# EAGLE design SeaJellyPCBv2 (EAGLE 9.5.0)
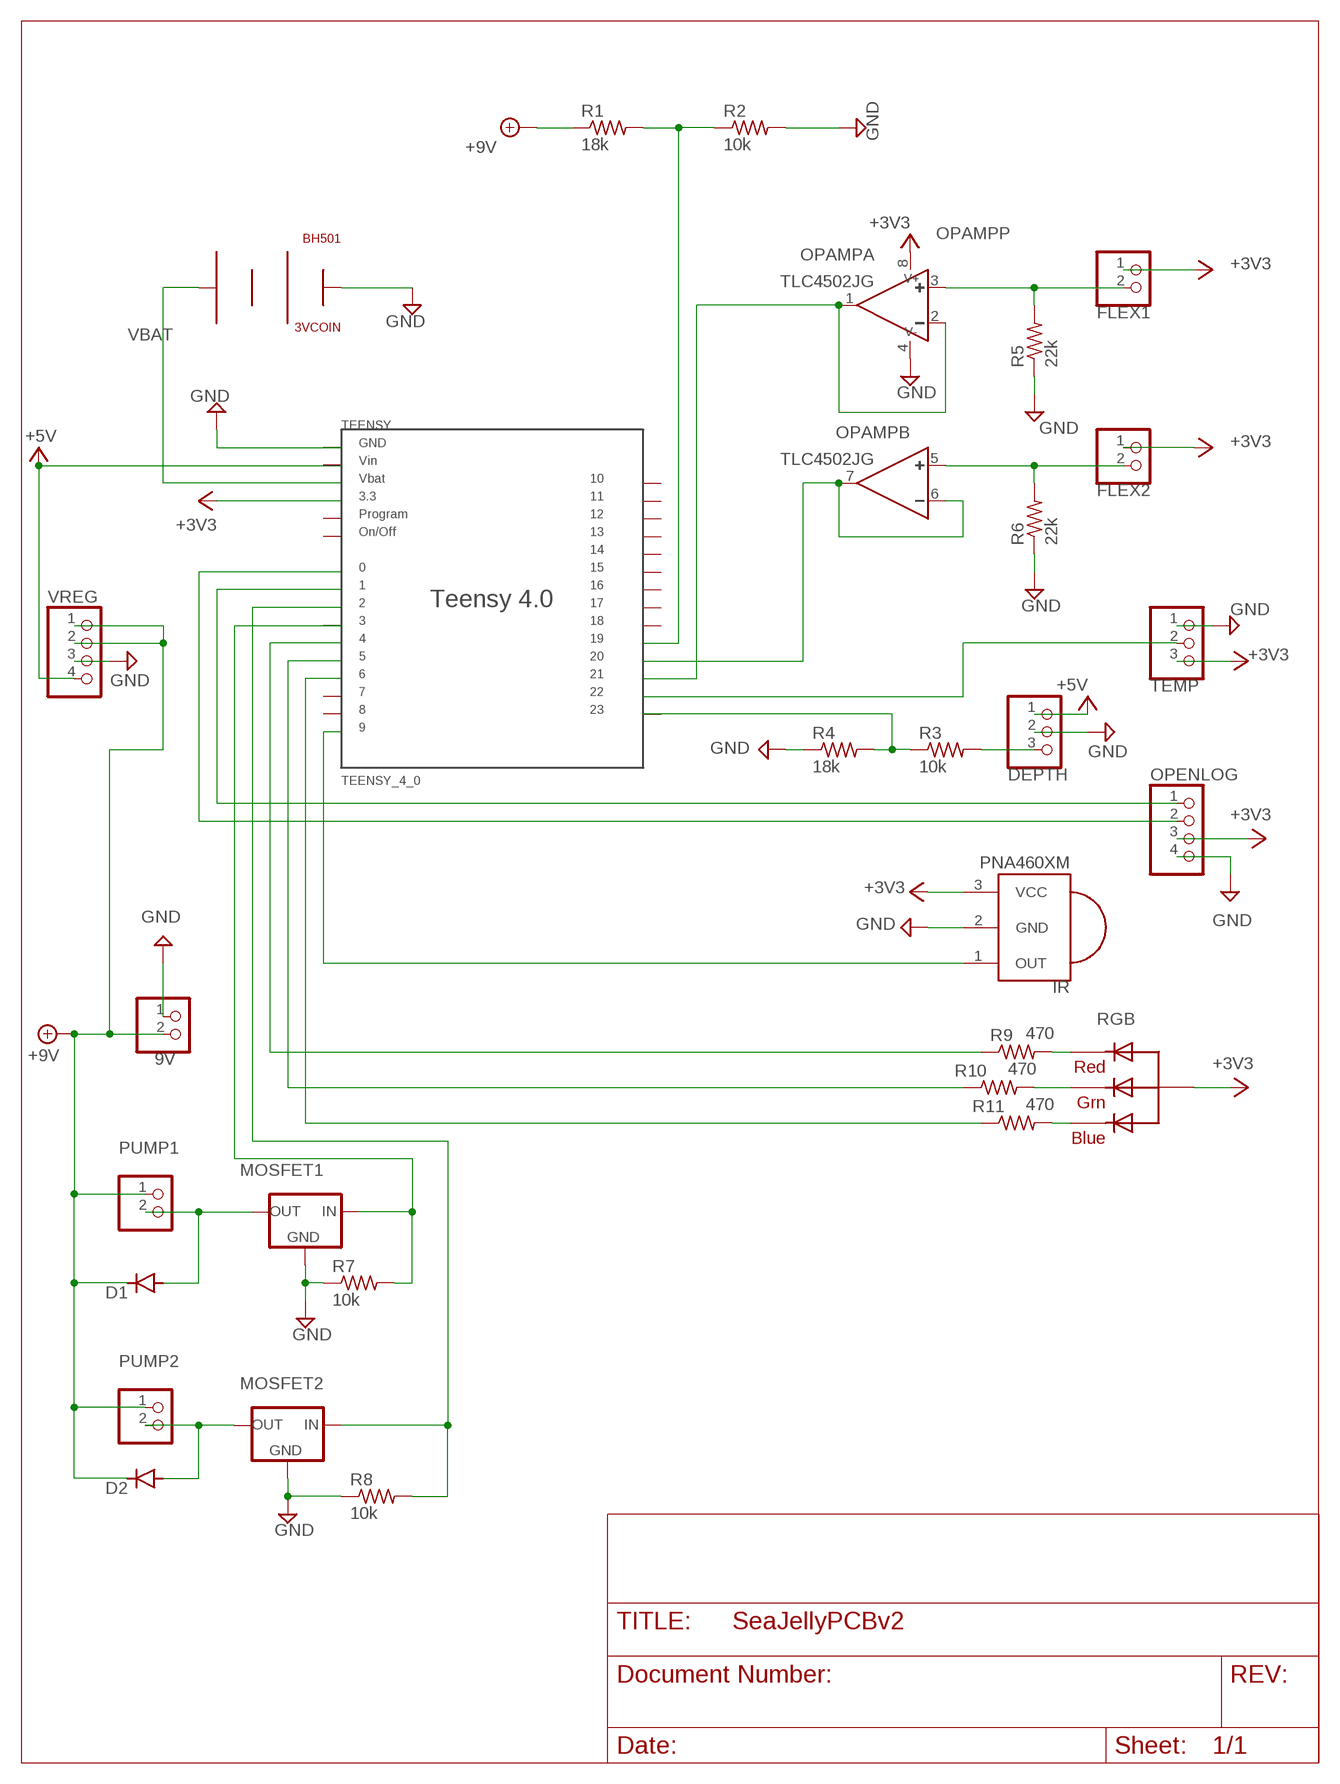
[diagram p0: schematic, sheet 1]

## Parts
3VCOIN  BH501  [BH501]
9V  PINHD-1X2  [1X02]
D1  DIODE-D-7.5  [D-7.5]
D2  DIODE-D-7.5  [D-7.5]
DEPTH  PINHD-1X3  [1X03]
FLEX1  PINHD-1X2  [1X02]
FLEX2  PINHD-1X2  [1X02]
IR  PNA460XM  [PNA460XM]
MOSFET1  MCP1700INLINE  [TO92-INLINE]
MOSFET2  MCP1700INLINE  [TO92-INLINE]
OPAMP  TLC4502JG  [DIL08]
OPENLOG  PINHD-1X4  [1X04]
PUMP1  PINHD-1X2  [1X02]
PUMP2  PINHD-1X2  [1X02]
R1  18k  R-US_0411/3V  [0411V]
R2  10k  R-US_0411/3V  [0411V]
R3  10k  R-US_0411/3V  [0411V]
R4  18k  R-US_0411/3V  [0411V]
R5  22k  R-US_0411/3V  [0411V]
R6  22k  R-US_0411/3V  [0411V]
R7  10k  R-US_0411/3V  [0411V]
R8  10k  R-US_0411/3V  [0411V]
R9  470  R-US_0411/3V  [0411V]
R10  470  R-US_0411/3V  [0411V]
R11  470  R-US_0411/3V  [0411V]
RGB  RGBLED_CA-5MM  [LED5MMRGB]
TEENSY  TEENSY_4_0  [TEENSY_4_0]
TEMP  PINHD-1X3  [1X03]
VREG  PINHD-1X4  [1X04]

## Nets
+3V3: FLEX1.1 FLEX2.1 IR.3(VCC) OPAMP.8(P:V+) OPENLOG.3 RGB.2(VCC) TEENSY.P$3_3_1(P$3_3) TEENSY.P$3_3_2(P$3_3) TEMP.3
+5V: DEPTH.1 TEENSY.P$VIN VREG.4
+9V [Power]: 9V.2 D1.C D2.C PUMP1.1 PUMP2.1 R1.1 VREG.1 VREG.2
DRAIN1 [Drain]: D1.A MOSFET1.3(OUT) PUMP1.2
DRAIN2 [Drain]: D2.A MOSFET2.3(OUT) PUMP2.2
GND [Ground]: 3VCOIN.P$NEG 9V.1 DEPTH.2 IR.2(GND) MOSFET1.1(GND) MOSFET2.1(GND) OPAMP.4(P:V-) OPENLOG.4 R2.2 R4.1 R5.1 R6.1 R7.1 R8.1 TEENSY.P$G1(P$GND) TEENSY.P$G2(P$GND) TEENSY.P$G3(P$GND) TEMP.1 VREG.3
N$1: R3.1 R4.2 TEENSY.P$23
N$2: OPAMP.6(B:-) OPAMP.7(B:OUT) TEENSY.P$20
N$3: MOSFET1.2(IN) R7.2 TEENSY.P$3
N$4: FLEX2.2 OPAMP.5(B:+) R6.2
N$5: FLEX1.2 OPAMP.3(A:+) R5.2
N$6: OPAMP.1(A:OUT) OPAMP.2(A:-) TEENSY.P$21
N$7: TEENSY.P$22 TEMP.2
N$8: DEPTH.3 R3.2
N$9: OPENLOG.1 TEENSY.P$1
N$10: OPENLOG.2 TEENSY.P$0
N$11: R11.2 RGB.4(BLUE)
N$12: R10.2 RGB.3(GREEN)
N$13: R9.1 TEENSY.P$4
N$14: R11.1 TEENSY.P$6
N$15: R9.2 RGB.1(RED)
N$16: R10.1 TEENSY.P$5
N$17: IR.1(OUT) TEENSY.P$9
N$19: MOSFET2.2(IN) R8.2 TEENSY.P$2
N$21: R1.2 R2.1 TEENSY.P$19
VBAT: 3VCOIN.P$POS TEENSY.P$VBAT
Unconnected: TEENSY.P$1/0 TEENSY.P$7 TEENSY.P$8 TEENSY.P$10 TEENSY.P$11 TEENSY.P$12 TEENSY.P$13 TEENSY.P$14 TEENSY.P$15 TEENSY.P$16 TEENSY.P$17 TEENSY.P$18 TEENSY.P$PROG(P$PGM)

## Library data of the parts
3VCOIN = BR1225:BH501
9V FLEX1 FLEX2 PUMP1 PUMP2 = pinhead:PINHD-1X2: PIN HEADER
D1 D2 = diode:DIODE-: DIODE
DEPTH TEMP = pinhead:PINHD-1X3: PIN HEADER
IR = adafruit:PNA460XM: IR 38KHz receiver PNA4602 and related receivers http://www.ladyada.net/library/pcb/eaglelibrary.html
MOSFET1 MOSFET2 = adafruit:MCP1700: VOLTAGE REGULATOR
OPAMP = texas:TLC4502: FAMILY OF SELF-CALIBRATING (Self-Cal TM) PRECISION CMOS RAIL-TO-RAIL OUTPUT OPERATIONAL AMPLIFIERS Source: Data sheet
OPENLOG VREG = pinhead:PINHD-1X4: PIN HEADER
R1-R11 = rcl:R-US_: RESISTOR, American symbol; SPICEPREFIX: R
RGB = adafruit:RGBLED_CA: RGB LED, common-anode 5MM Staggered pins 5mm Piranha package http://www.ladyada.net/library/pcb/eaglelibrary.html
TEENSY = Teensy_4_0:TEENSY_4_0

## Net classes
1 Ground: width 0.305 mm
2 Power: width 0.305 mm
3 Drain: width 0.305 mm

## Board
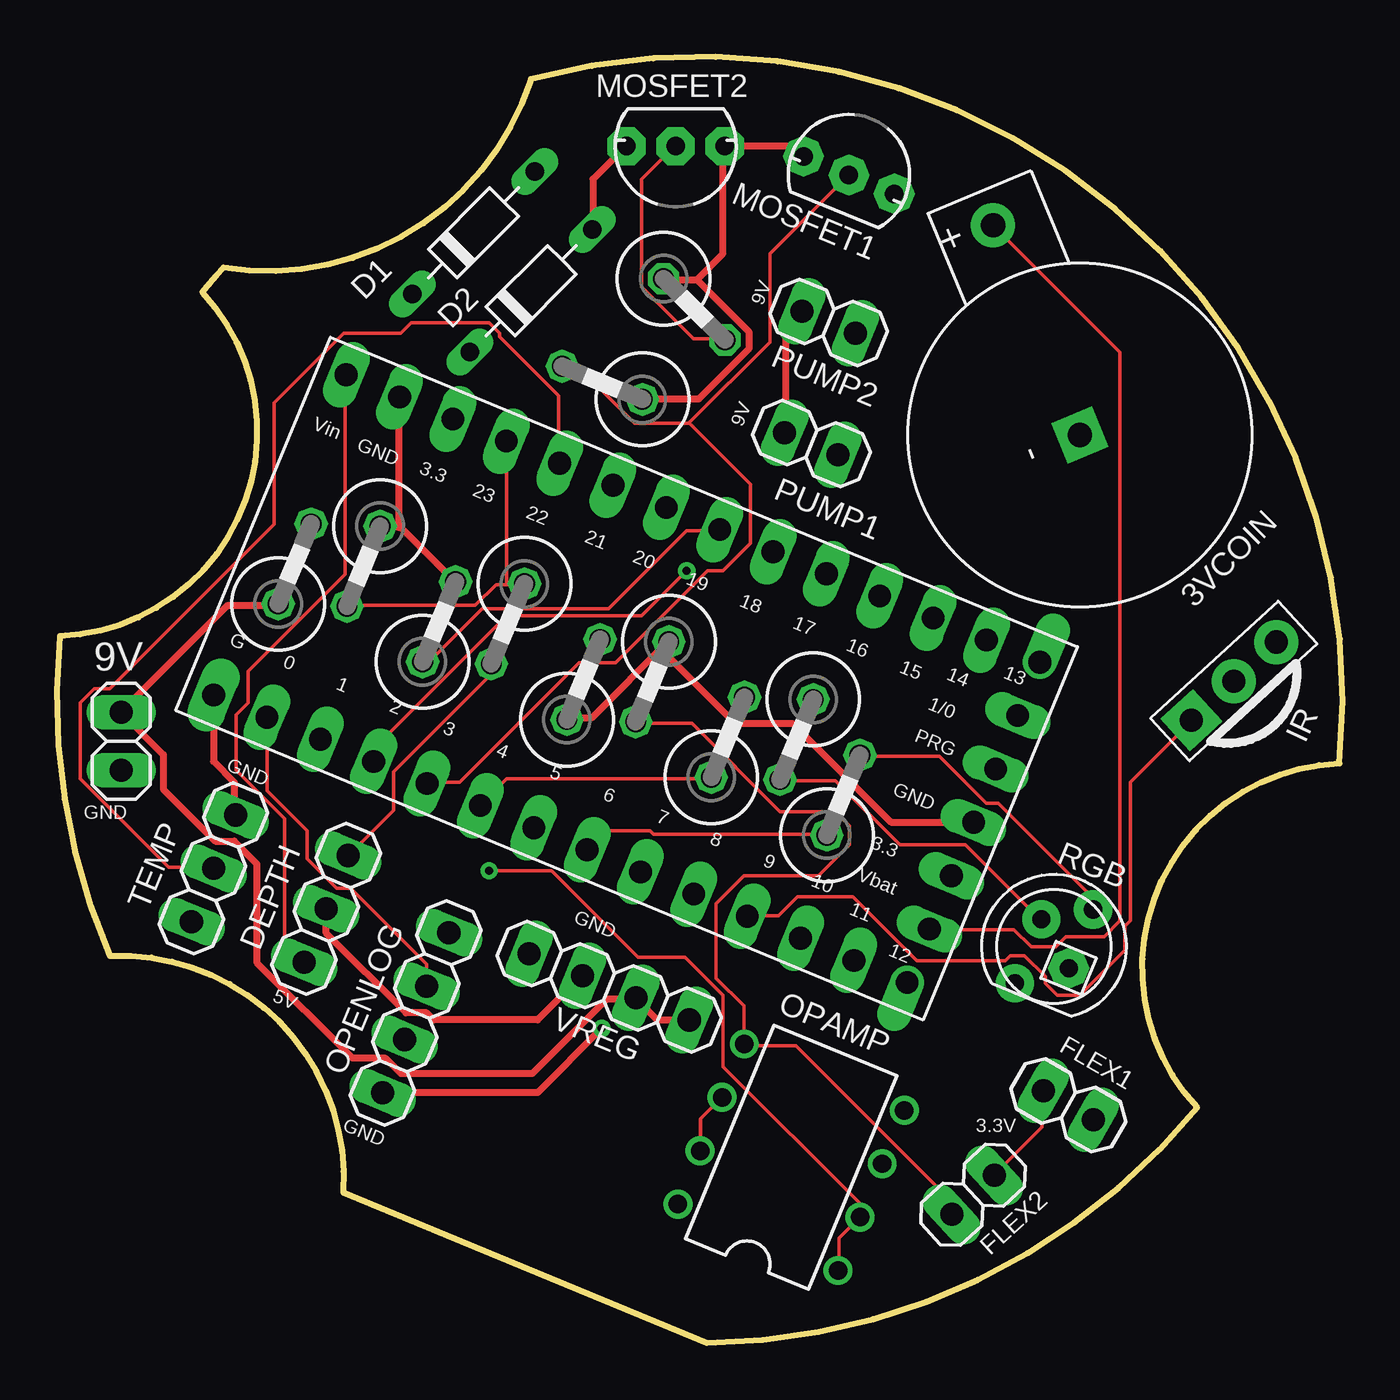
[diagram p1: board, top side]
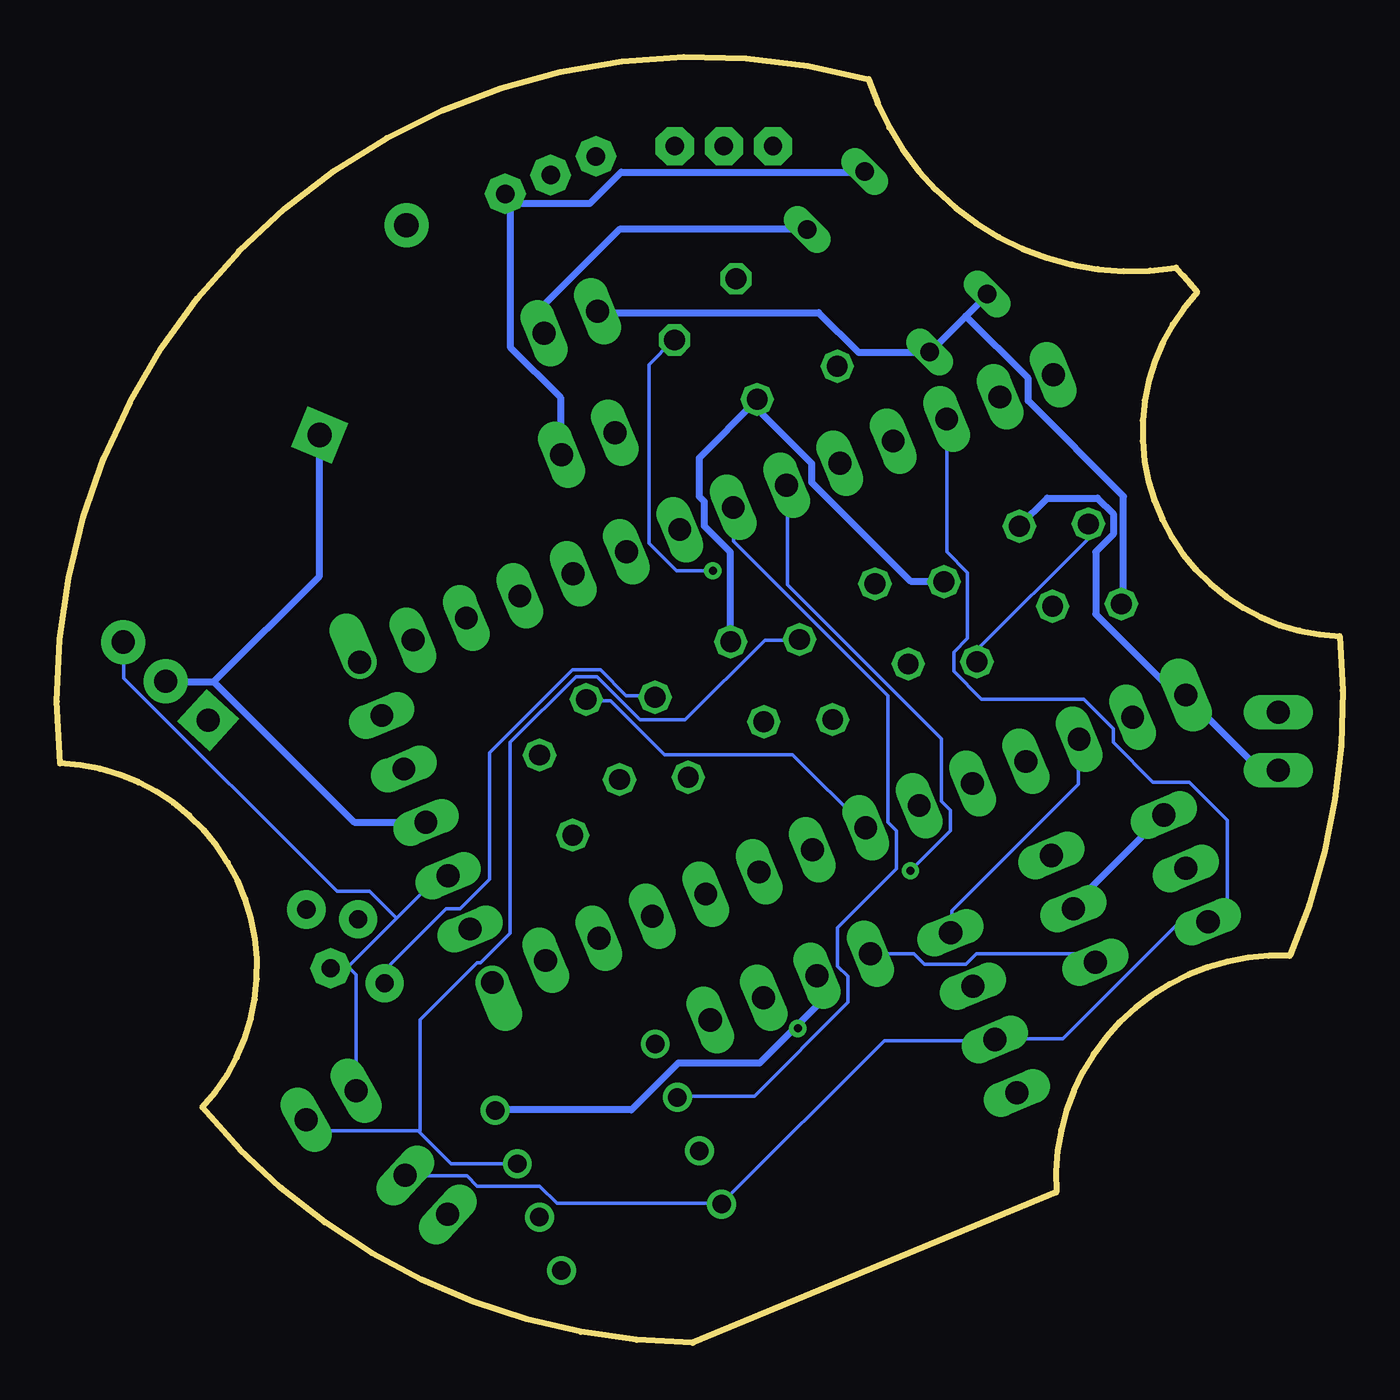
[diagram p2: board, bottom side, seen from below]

Size 56.55 x 56.54 mm. Coordinates in mm from the lower left corner, seen from the top.
Outline: 0.14,31.07 arc29 2.33,17.02 arc-96 12.59,6.62 28.59,0 arc50 50.14,10.36 arc-131 56.41,25.48 arc111 20.85,55.55 arc-81 7.33,47.27 arc3 6.4,46.19 arc-131 0.14,31.07
Copper layers (1*16): Top 0.0178mm / dielectric 59mil / Bottom 0.0178mm
Design rules "SSC-EAGLE-2Lyr_v1.0.0.3": minimum track width 6mil, minimum drill 14mil, track to track 6mil, track to pad 6mil, pad to pad 6mil, via to via 6mil, smd to smd 6mil, copper to edge 20mil, drill to drill 16mil, minimum pad ring 8mil, minimum via ring 8mil, stop-mask expansion 3mil, vias tented up to drill 0mil, thermal gap 10mil

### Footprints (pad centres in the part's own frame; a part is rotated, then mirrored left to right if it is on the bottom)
BH501 = drill 1.067 pad 1.93 square: P$NEG 0,0 | drill 1.067 pad 1.93: P$POS 9.982,0
1X02 = drill 1.016 long: 1 -1.27,0; 2 1.27,0
D-7.5 = drill 0.813 long: A 3.81,0; C -3.81,0
1X03 = drill 1.016 long: 1 -2.54,0; 2 0,0; 3 2.54,0
PNA460XM = drill 1.016 pad 1.93 square: 1 -2.54,0 | drill 1.016 pad 1.93: 2 0,0; 3 2.54,0
TO92-INLINE = drill 0.813 pad 1.676 octagon: 1 -2.159,0; 2 0,0; 3 2.159,0
DIL08 = drill 0.813 pad 1.27: 1 -3.81,-3.81; 2 -1.27,-3.81; 3 1.27,-3.81; 4 3.81,-3.81; 5 3.81,3.81; 6 1.27,3.81; 7 -1.27,3.81; 8 -3.81,3.81
1X04 = drill 1.016 long: 1 -3.81,0; 2 -1.27,0; 3 1.27,0; 4 3.81,0
0411V = drill 0.914 octagon: 1 -2.54,0; 2 1.27,0
LED5MMRGB = drill 0.8 pad 1.676: 1 -2.159,0.968; 3 0.889,0.968; 4 2.159,-0.968 | drill 0.8 pad 1.676 octagon: 2 -0.635,-0.968
TEENSY_4_0 = drill 1 long: P$0 2.54,0; P$1 5.08,0; P$1/0 33.02,12.7; P$2 7.62,0; P$3 10.16,0; P$3_3_1 5.08,15.24; P$3_3_2 33.02,5.08; P$4 12.7,0; P$5 15.24,0; P$6 17.78,0; P$7 20.32,0; P$8 22.86,0; P$9 25.4,0; P$10 27.94,0; P$11 30.48,0; P$14 30.48,15.24; P$15 27.94,15.24; P$16 25.4,15.24; P$17 22.86,15.24; P$18 20.32,15.24; P$19 17.78,15.24; P$20 15.24,15.24; P$21 12.7,15.24; P$22 10.16,15.24; P$23 7.62,15.24; P$G2 2.54,15.24; P$G3 33.02,7.62; P$PROG 33.02,10.16; P$VBAT 33.02,2.54; P$VIN 0,15.24 | drill 1 offset: P$12 33.02,0; P$13 33.02,15.24 | drill 1 pad 1.676 long: P$G1 0,0

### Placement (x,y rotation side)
3VCOIN  44.99,39.91 112.5 top
9V  2.83,26.45 90 top
D1  18.32,48.8 45 top
D2  20.86,46.26 45 top
DEPTH  11.84,19.09 67.5 top
FLEX1  44.48,10.45 330 top
FLEX2  40.29,6.51 222.5 top
IR  51.76,29.1 42.5 top
MOSFET1  34.83,51.34 337.5 top
MOSFET2  27.21,52.61 180 top
OPAMP  32.29,8.16 67.5 top
OPENLOG  15.78,14.51 247.5 top
PUMP1  33.18,39.53 337.5 top
PUMP2  33.94,44.87 337.5 top
R1  10.7,34.83 67.5 top
R2  17.05,32.29 67.5 top
R3  19.59,31.02 247.5 top
R4  13.24,33.56 247.5 top
R5  23.4,29.75 67.5 top
R6  25.94,28.48 247.5 top
R7  23.4,42.45 157.5 top
R8  28.48,44.99 315 top
R9  29.75,27.21 67.5 top
R10  32.29,25.94 247.5 top
R11  34.83,24.67 67.5 top
RGB  43.85,17.43 67.5 top
TEENSY  6.89,28.48 337.5 top
TEMP  6.89,20.86 247.5 top
VREG  24.29,15.66 157.5 top

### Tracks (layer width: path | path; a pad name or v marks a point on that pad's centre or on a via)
+3V3
  Top 0.152: FLEX1.1 43.32,11.08 43.32,9.48 41.26,7.43 FLEX2.1
  Bottom 0.152: TEENSY.P$3_3_1 17.41,40.57 17.41,34.78 16.49,33.87 16.49,30.97 17.1,30.36 17.1,29.52 15.88,28.3 11.39,28.3 10.09,27.01 10.09,26.4 8.34,24.65 6.74,24.65 5.06,22.97 5.06,19.39 5.9,18.55 TEMP.3 5.98,18.48 7.2,18.48 12.3,13.37 15.27,13.37 OPENLOG.3 15.35,13.29 20.15,13.29 27.31,6.13 OPAMP.8 27.39,6.13 34.55,6.13 35.31,6.89 38.06,6.89 38.51,7.35 41.18,7.35 FLEX2.1 | 41.6,18.67 43.77,16.49 44.46,16.49 RGB.2 43.7,16.49 43.39,16.19 FLEX1.1 | 41.6,18.67 39.73,20.53 39.35,20.53 TEENSY.P$3_3_2 | 41.6,18.67 42.78,19.85 44.23,19.85 53.6,29.22 53.6,30.74 IR.3
+5V
  Top 0.152: TEENSY.P$VIN 12.68,42.55 12.68,33.79 8.42,29.52 8.42,28.15 7.88,27.62 7.88,25.18 10.02,23.05 10.02,17.64 10.85,16.8 DEPTH.1
  Bottom 0.152: VREG.4 20.76,17.1 18.85,17.1 18.4,16.65 16.57,16.65 16.11,17.1 11.23,17.1 10.93,16.8 DEPTH.1
+9V
  Top 0.305: PUMP1.1 32.04,40.04 32.04,44.61 32.72,45.3 PUMP2.1 | VREG.1 27.77,14.21 26.4,14.21 25.48,15.12 VREG.2 25.33,15.12 24.19,15.12 20.91,11.85 15.12,11.85 14.44,12.53 12.99,12.53 8.8,16.72 8.8,21.07 7.81,22.06 6.97,22.06 4.68,24.34 4.68,25.87 9V.2 2.85,27.77 7.5,32.42 9.71,32.42 R1.1
  Bottom 0.305: 16.57,45.15 18.09,43.62 D2.C 18.32,43.55 21.29,43.55 23.05,45.3 32.72,45.3 PUMP2.1 | 16.57,45.15 15.65,46.06 D1.C | 16.57,45.15 13.83,42.4 13.83,41.41 9.63,37.22 9.63,32.57 9.71,32.5 R1.1
DRAIN1
  Bottom 0.305: D1.A 21.06,51.47 31.73,51.47 33.1,50.1 36.38,50.1 36.76,50.48 MOSFET1.3 36.46,50.02 36.61,49.87 36.61,43.77 34.4,41.56 34.4,39.05 PUMP1.2
DRAIN2
  Top 0.305: D2.A 23.58,49.03 23.58,51.17 25.03,52.61 MOSFET2.3
  Bottom 0.305: PUMP2.2 35.09,44.38 35.09,45.68 31.81,48.96 23.58,48.96 D2.A
GND  (via drill 0.36)
  Top 0.305: TEENSY.P$G1 6.89,25.56 7.81,24.65 7.81,23.28 TEMP.1 | v23.96,13.83 21.14,11.01 14.36,11.01 OPENLOG.4 | DEPTH.2 11.84,18.02 15.35,14.51 16.26,14.51 16.57,14.21 21.14,14.21 23.05,16.11 VREG.3 | 15.04,35.85 15.12,35.85 17.48,33.49 R2.2 | 15.04,35.85 14.28,35.85 R4.1 | 15.04,35.85 15.04,41.56 TEENSY.P$G2 | R5.1 22.44,27.47 23.5,27.47 26.86,30.82 R6.1 26.63,30.44 29.83,27.24 32.34,27.24 36.69,22.89 40.27,22.89 TEENSY.P$G3 | MOSFET1.1 32.8,52.23 32.42,52.61 MOSFET2.1 29.29,52.54 29.29,47.89 28.15,46.75 | 28.15,46.75 30.44,44.46 30.44,43.7 28.23,41.49 25.79,41.49 R7.1 | 28.15,46.75 26.7,46.75 R8.1
  Bottom 0.305: DEPTH.2 11.84,19.24 7.88,23.2 TEMP.1 | 9V.1 3.61,25.18 6.89,28.46 TEENSY.P$G1 6.97,28.61 7.42,28.61 10.85,32.04 10.85,34.78 10.09,35.54 10.09,36.46 10.78,37.14 12.99,37.14 14.21,35.93 R4.1 | 24.04,13.9 23.12,14.82 23.12,16.11 VREG.3 | 24.04,13.9 25.64,12.3 29.22,12.3 31.28,10.25 37.22,10.25 OPAMP.4 | v23.96,13.83 24.04,13.9 | 49.64,29.07 43.47,22.89 40.34,22.89 TEENSY.P$G3 | 49.64,29.07 51.7,29.07 51.77,29.14 IR.2 | 3VCOIN.P$NEG 44.99,33.72 49.64,29.07 | R6.1 26.93,30.9 26.93,34.78 28.08,35.93 28.08,36.99 28.3,37.22 28.3,38.9 25.79,41.41 R7.1 25.87,41.18 23.35,38.67 23.35,37.83 19.01,33.49 17.56,33.49 R2.2
N$1
  Top 0.152: 19.77,33.33 20.53,33.33 R3.1 | 19.77,33.33 19.31,33.33 18.4,32.42 12.76,32.42 R4.2 | 19.77,33.33 19.77,39.58 TEENSY.P$23
N$2
  Top 0.152: OPAMP.7 28.3,8.49 28.3,9.87 29.22,10.78 OPAMP.6
  Bottom 0.152: TEENSY.P$20 26.78,36.69 26.78,35.24 20,28.46 20,22.89 19.62,22.51 19.62,20.84 22.21,18.25 22.21,16.57 21.75,16.11 21.75,14.97 25.87,10.86 29.22,10.86 OPAMP.6
N$3
  Top 0.152: 27.81,40.46 31.35,44 31.35,47.89 34.78,51.32 MOSFET1.2 | 27.81,40.46 27.77,40.42 25.41,40.42 22.89,42.94 22.28,42.94 R7.2 | 27.81,40.46 30.51,37.75 30.51,35.16 29.29,33.94 28.61,33.94 24.57,29.91 22.97,29.91 17.71,24.65 16.34,24.65 TEENSY.P$3
N$4
  Top 0.152: FLEX2.2 39.35,5.67 39.35,6.21 32.49,13.06 30.28,13.06 OPAMP.5 30.21,13.22 30.21,14.82 28.99,16.04 28.99,19.31 30.21,20.53 33.49,20.53 34.86,21.9 34.86,22.74 34.25,23.35 31.81,23.35 27.92,27.24 25.48,27.24 R6.2
N$5
  Bottom 0.152: 40.61,9.29 40.65,9.33 45.07,9.33 45.52,9.79 FLEX1.2 | 40.61,9.29 39.2,7.88 OPAMP.3 | R5.2 23.96,30.9 25.41,30.9 28.91,27.39 30.89,27.39 32.8,29.3 33.71,29.3 36.61,26.4 36.61,18.02 37.9,16.72 38.06,16.72 40.57,14.21 40.57,9.33 40.61,9.29
N$6  (via drill 0.36)
  Top 0.152: OPAMP.1 34.4,3.24 34.4,4.61 35.31,5.52 OPAMP.2 35.31,5.6 35.31,6.13 29.29,12.15 29.29,15.27 27.62,16.95 25.56,16.95 21.75,20.76 v19.01,20.76
  Bottom 0.152: v19.01,20.76 17.25,22.51 17.25,23.43 17.64,23.81 17.64,26.55 24.42,33.33 24.42,37.68 TEENSY.P$21
N$7
  Top 0.152: TEENSY.P$22 22.06,38.75 22.06,41.64 19.46,44.23 19.46,44.38 19.01,44.84 15.58,44.84 15.12,44.38 12.61,44.38 9.56,41.34 9.56,36 2.32,28.76 1.63,28.76 1.02,28.15 1.02,24.8 4.91,20.91 6.89,20.91 TEMP.2
N$8
  Top 0.152: R3.2 19.08,29.83 19.08,29.37 14.82,25.11 14.82,23.43 12.84,21.45 DEPTH.3
N$9
  Bottom 0.152: TEENSY.P$1 11.62,26.48 11.62,24.57 17.18,19.01 17.18,18.09 OPENLOG.1
N$10
  Top 0.152: TEENSY.P$0 9.25,27.47 9.25,24.27 11.01,22.51 11.01,21.29 12.3,20 12.91,20 16.26,16.65 16.26,15.73 OPENLOG.2
N$11
  Top 0.152: R11.2 35.39,25.79 38.82,25.79 40.88,23.73 41.41,23.73 45.52,19.62 45.52,19.09 RGB.4
N$12
  Top 0.152: R10.2 31.81,24.72 34.25,24.72 37.07,21.9 39.96,21.9 43.24,18.63 RGB.3
N$13
  Top 0.152: R9.1 28.76,24.8 19.77,24.8 18.63,23.66 TEENSY.P$4
N$14
  Top 0.152: R11.1 33.79,22.36 26.25,22.36 26.09,22.51 24.11,22.51 23.35,21.75 TEENSY.P$6
N$15
  Bottom 0.152: R9.2 30.28,28.46 31.5,28.46 32.65,29.6 33.87,29.6 37.52,25.94 37.52,20.38 38.82,19.09 39.43,19.09 42.1,16.42 42.1,15.88 RGB.1
N$16
  Bottom 0.152: R10.1 33.26,28.23 32.19,28.23 29.83,25.87 24.19,25.87 20.99,22.67 TEENSY.P$5
N$17
  Top 0.152: TEENSY.P$9 30.36,18.78 31.73,18.78 32.57,19.62 35.01,19.62 37.83,16.8 41.71,16.8 41.94,17.03 42.55,17.03 43.47,16.11 43.47,15.81 44,15.27 44.99,15.27 46.97,17.26 46.97,18.32 47.2,18.55 47.2,24.65 49.87,27.32 IR.1
N$19  (via drill 0.36)
  Top 0.152: R8.2 29.37,44.16 28,44.16 25.71,46.44 25.71,51.17 27.16,52.61 MOSFET2.2 | v27.69,33.94 25.71,31.96 19.77,31.96 13.98,26.17 13.98,25.64 TEENSY.P$2
  Bottom 0.152: v27.69,33.94 29.29,33.94 30.51,35.16 30.51,43.01 29.45,44.08 R8.2
N$21
  Top 0.152: TEENSY.P$19 29.14,35.7 27.69,35.7 24.27,32.27 18.7,32.27 16.42,29.98 16.11,29.98 R2.1
  Bottom 0.152: R1.2 11.23,36 11.23,35.32 16.04,30.52 16.04,29.98 R2.1
VBAT
  Top 0.152: TEENSY.P$VBAT 38.44,18.17 42.1,18.17 42.86,17.41 43.92,17.41 44.38,17.87 46.06,17.87 46.74,18.55 46.74,43.55 41.18,49.11 3VCOIN.P$POS

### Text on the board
tPlace: 9V | 9V | GND | GND | GND | 5V | 3.3V | GND
tNames: IR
